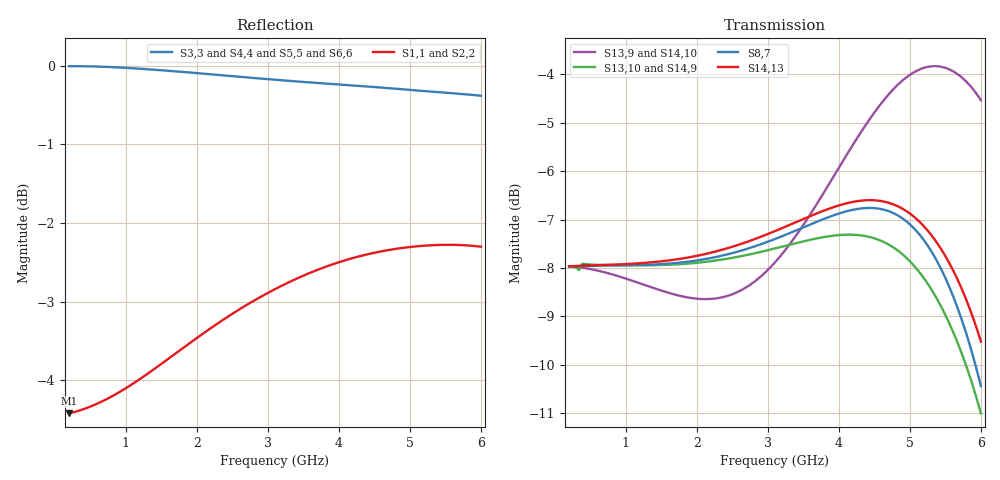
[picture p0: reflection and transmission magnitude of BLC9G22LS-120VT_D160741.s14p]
! Touchstone file from project EMMA_Start_Packages
! Exported from HFSS 2014.0.7
! Variables:
!  AirBox_H = 45mm
!  AirBox_L = 40mm
!  AirBox_W = 140mm
!  Thinner = 21.4um
!  pcb_h = 760um
# GHZ S MA R 50.000000
! Terminal data exported
! Port[1] = 1DRF
! Port[2] = 1GRF
! Port[3] = 2DVT
! Port[4] = 2GVT
! Port[5] = 3DVD
! Port[6] = 3GVD
! Port[7] = P3_BWT4_Rect_T1
! Port[8] = P3_BWT4_Rect_1_T1
! Port[9] = P5_BWT5_7_Rect_T1
! Port[10] = P5_BWT5_7_Rect_1_T1
! Port[11] = P6_BWT2_3_Rect_T1
! Port[12] = P6_BWT2_3_Rect_1_T1
! Port[13] = P7_BWT6_Rect_T1
! Port[14] = P7_BWT6_Rect_1_T1
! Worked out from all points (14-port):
!   291 points, 200 MHz to 6 GHz, reference per port
!   strongest paths, dB at 200 MHz, 1.64 GHz, 3.1 GHz, 4.56 GHz, 6 GHz:
!     S14,13: -8.0, -7.8, -7.2, -6.6, -9.5
!     S8,7: -8.0, -7.9, -7.4, -6.8, -10.4
!     S13,10: -8.0, -7.9, -7.6, -7.4, -11.0
!     S14,9: -8.0, -7.9, -7.6, -7.4, -11.0
!     S13,9: -8.0, -8.5, -7.9, -4.7, -4.5
!     S14,10: -8.0, -8.5, -7.9, -4.7, -4.5
!   lowest |S11| = -4.4 dB at 200 MHz (marker M1), VSWR 4.01
!   |S11| at or under -10 dB: nowhere
